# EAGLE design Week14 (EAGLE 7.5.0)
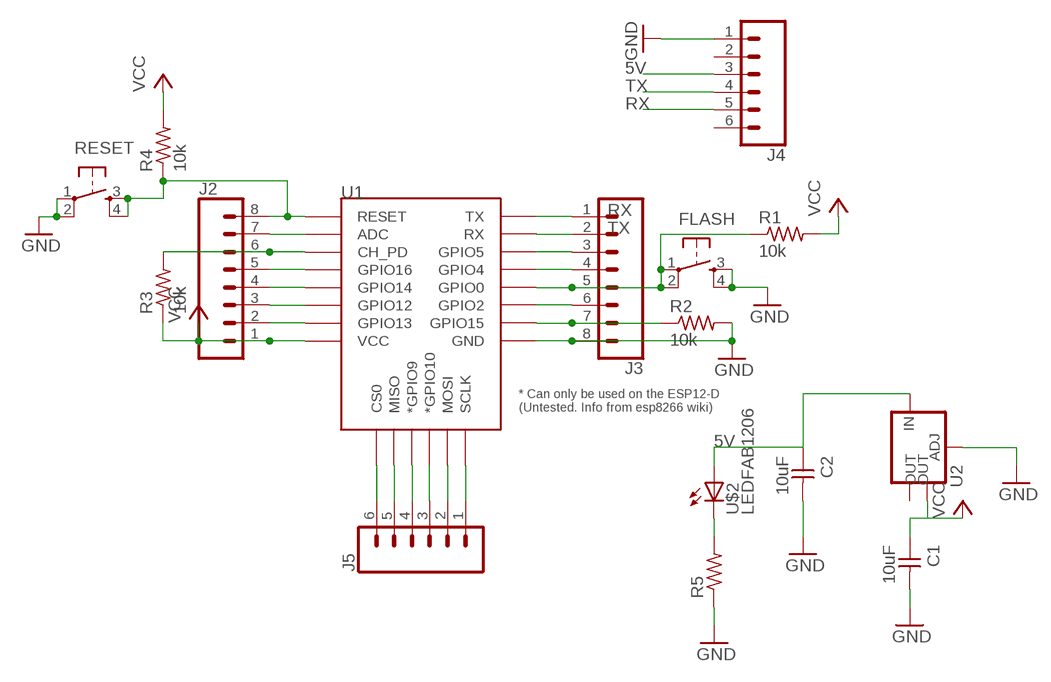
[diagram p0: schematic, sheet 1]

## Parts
C1  10uF  CAP-UNPOLARIZEDFAB  [C1206FAB]
C2  10uF  CAP-UNPOLARIZEDFAB  [C1206FAB]
FLASH  6MM_SWITCH6MM_SWITCH  [6MM_SWITCH]
J2  CONN_08"  [1X08]
J3  CONN_08"  [1X08]
J4  CONN_06SILK_FEMALE_PTH  [1X06]
J5  CONN_06SILK_FEMALE_PTH  [1X06]
R1  10k  RES-US1206FAB  [R1206FAB]
R2  10k  RES-US1206FAB  [R1206FAB]
R3  10k  RES-US1206FAB  [R1206FAB]
R4  10k  RES-US1206FAB  [R1206FAB]
R5  RES-US1206FAB  [R1206FAB]
RESET  6MM_SWITCH6MM_SWITCH  [6MM_SWITCH]
U1  ESP12ESMD  [ESP12E-SMD]
U2  V_REG_LM1117SOT223  [SOT223]
U$2  LEDFAB1206  [LED1206FAB]

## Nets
5V: C2.1 J4.3 U2.3(IN) U$2.1(A)
GND: C1.2 C2.2 FLASH.3(S) FLASH.4(S1) J3.8 J4.1 R2.2 R5.1 RESET.1(P) RESET.2(P1) U1.GND U2.1(ADJ)
N$1: J5.6 U1.CS0
N$2: J5.5 U1.MISO
N$3: J5.4 U1.GPIO9(*GPIO9)
N$4: J5.3 U1.GPIO10(*GPIO10)
N$5: J5.2 U1.MOSI
N$6: J5.1 U1.SCLK
N$7: FLASH.1(P) FLASH.2(P1) J3.5 R1.1 U1.GPIO0
N$9: J3.3 U1.GPIO5
N$10: J3.4 U1.GPIO4
N$12: J3.6 U1.GPIO2
N$13: J3.7 R2.1 U1.GPIO15
N$14: J2.5 U1.GPIO16
N$15: J2.8 R4.1 RESET.3(S) RESET.4(S1) U1.RESET
N$16: J2.7 U1.ADC
N$17: J2.6 R3.2 U1.CH_PD
N$18: J2.4 U1.GPIO14
N$19: R5.2 U$2.2(C)
N$20: J2.3 U1.GPIO12
N$21: J2.2 U1.GPIO13
RX: J3.1 J4.5 U1.TXD0(TX)
TX: J3.2 J4.4 U1.RXD0(RX)
VCC: C1.1 J2.1 R1.2 R3.1 R4.2 U1.VCC U2.4(OUT)
Unconnected: J4.2 J4.6 U2.2(OUT)

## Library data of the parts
C1 C2 = fab:CAP-UNPOLARIZED
FLASH RESET = fab:6MM_SWITCH: OMRON SWITCH
J2 J3 = SparkFun-Connectors:CONN_08: Multi connection point. Often used as Generic Header-pin footprint for 0.1 inch spaced/style header connections On any of the 0.1 inch spaced packages, you can populate with these: Break Away Headers - Straight (PRT-00116) Break Away Male Headers - Right Angle (PRT-00553) Female Headers (PRT-00115)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; PROD_ID: CONN-08438
J4 J5 = SparkFun-Connectors:CONN_06: Multi connection point. Often used as Generic Header-pin footprint for 0.1 inch spaced/style header connections On any of the 0.1 inch spaced packages, you can populate with these: Break Away Headers - Straight (PRT-00116) Break Away Male Headers - Right Angle (PRT-00553) Female Headers (PRT-00115)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; PROD_ID: CONN-08437
R1-R5 = fab:RES-US: Resistor (US Symbol)
U1 = esp8266modules:ESP12E: ESP12E Module
U2 = SparkFun-IC-Power:V_REG_LM1117: Voltage Regulator LM1117 Standard adjustable voltage regulator but in SMD form. Spark Fun Electronics SKU : COM-00595; PROD_ID: VREG-08170
U$2 = fab:LED: LED

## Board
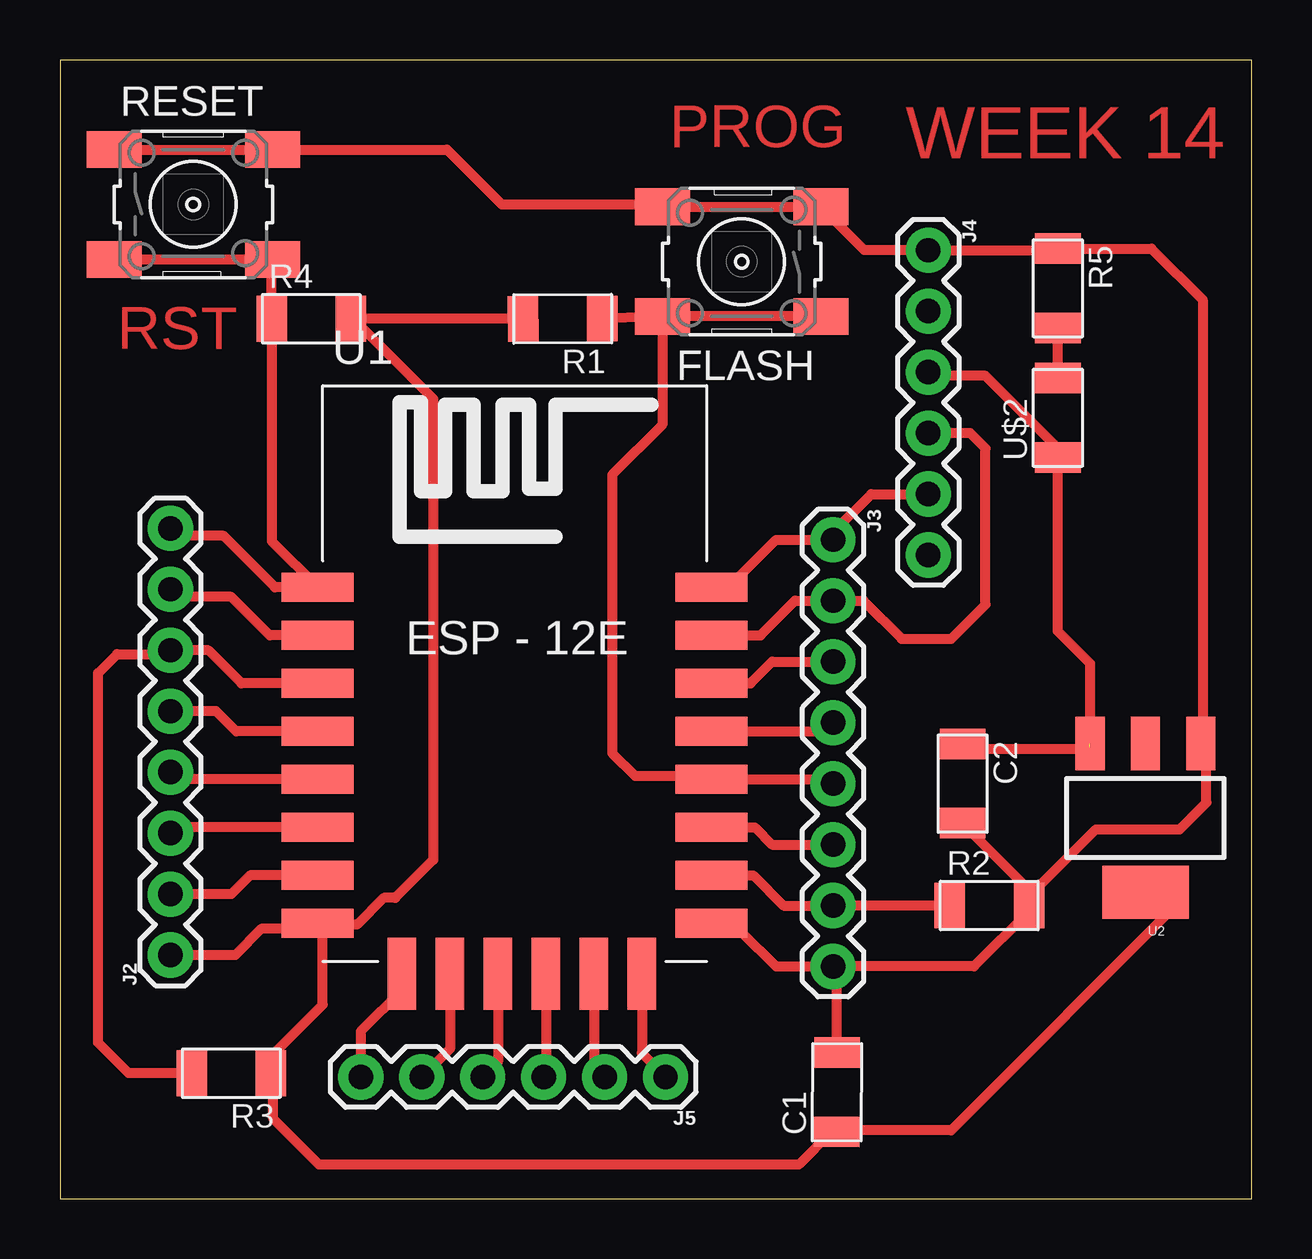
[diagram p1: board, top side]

Size 49.67 x 47.45 mm. Coordinates in mm from the lower left corner, seen from the top.
Outline: 0,0 49.67,0 49.67,47.45 0,47.45 0,0
Copper layers (1*16): Top 0.035mm / dielectric 1.5mm / Bottom 0.035mm
Design rules "default": minimum track width 10mil, minimum drill 24mil, track to track 8mil, track to pad 8mil, pad to pad 8mil, via to via 8mil, smd to smd 8mil, copper to edge 40mil, drill to drill 8mil, minimum pad ring 10mil, minimum via ring 8mil, stop-mask expansion 4mil, vias tented up to drill 0mil, thermal gap 10mil

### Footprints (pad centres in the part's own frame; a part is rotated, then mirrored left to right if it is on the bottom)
C1206FAB = smd 1.27 x 1.905: 1 -1.651,0; 2 1.651,0
6MM_SWITCH = smd 2.286 x 1.524: 1 -3.302,2.286; 2 3.302,2.286; 3 -3.302,-2.286; 4 3.302,-2.286
1X08 = drill 1.016 pad 1.88: 1 0,0; 2 2.54,0; 3 5.08,0; 4 7.62,0; 5 10.16,0; 6 12.7,0; 7 15.24,0; 8 17.78,0
1X06 = drill 1.016 pad 1.88: 1 0,0; 2 2.54,0; 3 5.08,0; 4 7.62,0; 5 10.16,0; 6 12.7,0
R1206FAB = smd 1.27 x 1.905: 1 -1.651,0; 2 1.651,0
ESP12E-SMD = smd 3 x 1.2: ADC -8.3,3.8; CH_PD -8.3,1.8; GND 8.1,-8.2; GPIO0 8.1,-2.2; GPIO2 8.1,-4.2; GPIO4 8.1,-0.2; GPIO5 8.1,1.8; GPIO12 -8.3,-4.2; GPIO13 -8.3,-6.2; GPIO14 -8.3,-2.2; GPIO15 8.1,-6.2; GPIO16 -8.3,-0.2; RESET -8.3,5.8; RXD0 8.1,3.8; TXD0 8.1,5.8; VCC -8.3,-8.2 | smd 1.2 x 3: CS0 -4.8,-10.3; GPIO9 -0.8,-10.3; GPIO10 1.2,-10.3; MISO -2.8,-10.3; MOSI 3.2,-10.3; SCLK 5.2,-10.3
SOT223 = smd 1.219 x 2.235: 1 -2.311,-3.099; 2 0,-3.099; 3 2.311,-3.099 | smd 3.6 x 2.2: 4 0,3.099
LED1206FAB = smd 1.27 x 1.905: 1 -1.651,0; 2 1.651,0

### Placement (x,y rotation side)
C1  32.39,4.45 89.8 top
C2  37.62,17.3 270 top
FLASH  28.42,39.05 180 top
J2  4.6,10.16 90 top
J3  32.23,27.46 270 top
J4  36.2,39.53 270 top
J5  25.24,5.08 180 top
R1  20.95,36.67 180.2 top
R2  38.73,12.22 0 top
R3  7.14,5.24 180 top
R4  10.48,36.67 0 top
R5  41.59,37.94 270 top
RESET  5.56,41.43 0 top
U1  19.05,19.68 0 top
U2  45.24,15.88 180 top
U$2  41.59,32.54 90 top

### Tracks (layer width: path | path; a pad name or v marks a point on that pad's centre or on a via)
5V  (1 unrouted)
  Top 0.406: 42.93,18.82 43.02,18.73 37.85,18.73 C2.1 | J4.3 36.35,34.29 38.58,34.29 41.59,31.27 U$2.1 41.59,23.65 42.93,22.31 U2.3 42.68,18.66
GND
  Top 0.406: FLASH.4 FLASH.3 33.53,39.53 J4.1 41.53,39.53 R5.1 45.5,39.59 47.63,37.47 47.63,19.05 47.94,18.73 47.94,18.57 47.78,18.41 | U1.GND 27.94,11.11 28.42,11.11 29.85,9.68 J3.8 | RESET.1 RESET.2 16.13,43.72 18.42,41.43 25.02,41.43 FLASH.4 | 25.11,41.18 FLASH.4 | C1.2 32.39,9.52 J3.8 | R2.2 40.39,11.97 38.1,9.68 J3.8 | R2.2 40.39,12.89 C2.2 | R2.2 40.39,12.61 43.18,15.4 46.67,15.4 47.78,16.51 47.78,18.41 | 47.78,18.41 47.78,18.75 U2.1
N$1
  Top 0.406: U1.CS0 14.25,8.69 12.54,6.99 J5.6 12.54,4.6
N$2
  Top 0.406: U1.MISO 16.25,6.25 J5.5
N$3
  Top 0.406: U1.GPIO9 18.25,5.71 J5.4
N$4
  Top 0.406: U1.GPIO10 20.25,5.17 J5.3
N$5
  Top 0.406: U1.MOSI 22.25,5.53 J5.2
N$6
  Top 0.406: U1.SCLK 24.25,6.07 J5.1
N$7
  Top 0.406: FLASH.1 FLASH.2 | FLASH.2 R1.1 | U1.GPIO0 28.1,17.48 | 28.1,17.48 32.05,17.48 J3.5 | FLASH.2 25.11,32.26 23.02,30.16 23.02,18.57 23.97,17.62 27.96,17.62 28.1,17.48
N$9
  Top 0.406: U1.GPIO5 28.79,21.48 29.69,22.38 J3.3
N$10
  Top 0.406: U1.GPIO4 31.87,19.48 J3.4
N$12
  Top 0.406: U1.GPIO2 28.97,15.48 29.69,14.76 J3.6
N$13
  Top 0.406: R2.1 J3.7 30.16,12.22 28.9,13.48 U1.GPIO15
N$14
  Top 0.406: U1.GPIO16 7.34,19.48 6.51,20.32 J2.5
N$15
  Top 0.406: U1.RESET 10.88,25.48 10.95,25.56 | RESET.3 RESET.4 8.83,39.12 R4.1 8.83,27.41 U1.RESET | U1.RESET 8.96,25.48 6.83,27.62 4.92,27.62 J2.8
N$16
  Top 0.406: U1.ADC 8.74,23.48 7.14,25.08 4.92,25.08 J2.7
N$17
  Top 0.406: U1.CH_PD 7.57,21.48 6.19,22.86 J2.6 4.45,22.7 2.38,22.7 1.59,21.91 1.59,6.51 2.86,5.24 R3.2
N$18
  Top 0.406: U1.GPIO14 4.9,17.48 J2.4
N$19
  Top 0.406: U$2.2 R5.2
N$20
  Top 0.406: U1.GPIO12 4.85,15.48 J2.3
N$21
  Top 0.406: U1.GPIO13 7.93,13.48 7.14,12.7 J2.2
RX
  Top 0.406: U1.TXD0 27.87,25.48 29.85,27.46 J3.1 32.23,27.78 33.81,29.37 J4.5
TX
  Top 0.406: U1.RXD0 29.2,23.48 30.64,24.92 J3.2 33.5,24.92 35.08,23.34 37.15,23.34 38.58,24.77 38.58,31.27 37.94,31.91 J4.4
VCC
  Top 0.406: U1.VCC 9.4,11.25 8.39,11.25 7.3,10.16 J2.1 | R1.2 R4.2 12.22,36.67 15.56,33.34 15.56,14.13 13.97,12.54 13.49,12.54 12.38,11.43 10.81,11.43 U1.VCC | U2.4 46.75,12.46 37.15,2.86 32.44,2.86 C1.1 32.16,2.79 30.8,1.43 10.8,1.43 8.89,3.33 8.89,5.14 R3.1 8.8,5.94 10.95,8.1 10.95,11.28 U1.VCC

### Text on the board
Top: PROG | WEEK 14 | RST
